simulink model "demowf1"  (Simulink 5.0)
settings: Solver=ode4  StartTime=0.0  StopTime=100  FixedStep=0.1  RelTol=1e-3
libraries: simulink_extras x5, MarineGNC x5, simulink x2

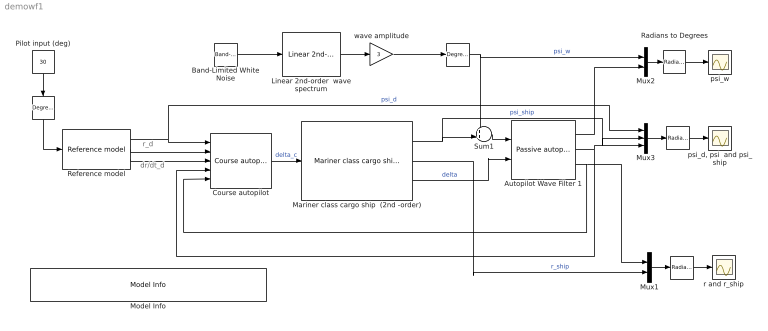
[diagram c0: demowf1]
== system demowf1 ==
  note: r_d
  note: dr/dt_d
  " " : simulink_extras/Transformations/Radians to Degrees
  "  " : simulink_extras/Transformations/Radians to Degrees
  "   " : simulink_extras/Transformations/Degrees to Radians
  "     " : simulink_extras/Transformations/Degrees to Radians  Orientation=down
  Autopilot Wave Filter 1 : MarineGNC/Navigation/Wave filters/Passive autopilot wave filter 1  lambda=0.1  w_o=1.2  K4=0.1  K5=0.01  w_c=1.3  T=107.3  K=0.185  T_b=100
  Band-Limited White Noise : simulink/Sources/Band-Limited White Noise  Cov=[1]  Ts=0.1  seed=[23341]
  Course autopilot : MarineGNC/Control/Ship control systems/Course autopilot  T_nomoto=107.3  K_nomoto=0.185  Kp=2  Td=50  Ti=100
  Linear 2nd-order  wave spectrum : MarineGNC/Models/Waves, wind and currents/Linear 2nd-order  wave spectrum  sigma=0.5  w_0=1.2  lambda=0.1
  Mariner class cargo ship  (2nd -order) : MarineGNC/Models/Vessels/Mariner class cargo ship  (2nd -order)  rate_max=5*(pi/180)  delta_max=20*(pi/180)  K=0.185  T1=118  T2=7.8  T3=18.5
  Model Info : simulink/Model-Wide Utilities/Model Info  InitialBlockCM=None  BlockCM=None  Frame=on  DisplayStringWithTags=|  HorizontalTextAlignment=Left  LeftAlignmentValue=0.02  SourceBlockDiagram=demowf1  TagMaxNumber=20
      | Autopilot demo using only compass measurements
      | %<Creator>Author: Thor I. Fossen
      | %<LastModificationDate>
  Mux1 : Mux  Inputs=2
  Mux2 : Mux  Inputs=2
  Mux3 : Mux  Inputs=3
  Pilot input (deg) : Constant  Orientation=down  Value=30
  "Radians to Degrees  " : simulink_extras/Transformations/Radians to Degrees
  Reference model : MarineGNC/Guidance/Reference model  v_max=1  zeta_d=1.0  w_d=0.1
  Sum1 : Sum  Inputs=++|
  "psi_d, psi  and psi_ship" : Scope
  psi_w : Scope
  r and r_ship : Scope
  wave amplitude : Gain  Gain=3
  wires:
  Band-Limited White Noise/1 -> Linear 2nd-order  wave spectrum/1
  Mux2/1 -> "Radians to Degrees  "/1
  "Radians to Degrees  "/1 -> psi_w/1
  " "/1 -> "psi_d, psi  and psi_ship"/1
  Mux1/1 -> "  "/1
  "  "/1 -> r and r_ship/1
  Linear 2nd-order  wave spectrum/1 -> wave amplitude/1
  Mux3/1 -> " "/1
  Mariner class cargo ship  (2nd -order)/3 -> Autopilot Wave Filter 1/2  "delta"
  wave amplitude/1 -> "   "/1
  Course autopilot/1 -> Mariner class cargo ship  (2nd -order)/1  "delta_c"
  Autopilot Wave Filter 1/2 -> Mux3/3, Course autopilot/4
  Autopilot Wave Filter 1/3 -> Mux1/1, Course autopilot/5
  Mariner class cargo ship  (2nd -order)/1 -> Sum1/2, Mux3/2  "psi_ship"
  Sum1/1 -> Autopilot Wave Filter 1/1
  "   "/1 -> Sum1/1, Mux2/1  "psi_w"
  Mariner class cargo ship  (2nd -order)/2 -> Mux1/2  "r_ship"
  Reference model/1 -> Mux3/1, Course autopilot/1  "psi_d"
  Reference model/2 -> Course autopilot/2
  Reference model/3 -> Course autopilot/3
  Autopilot Wave Filter 1/1 -> Mux2/2
  Pilot input (deg)/1 -> "     "/1
  "     "/1 -> Reference model/1
